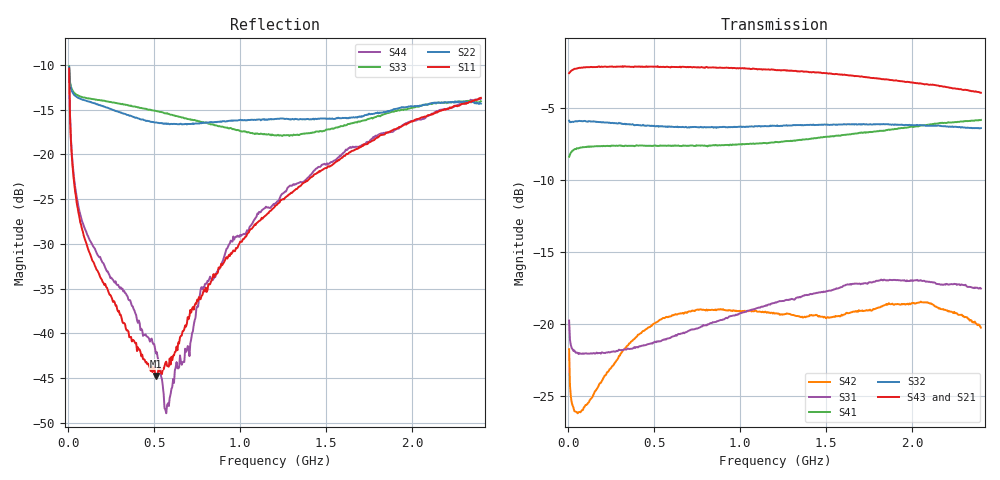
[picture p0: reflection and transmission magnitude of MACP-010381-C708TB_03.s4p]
!Agilent Technologies,E5071B,JP1KK00267,A.09.10
!Date: Mon Mar 23 11:06:01 2020
!Data & Calibration Information:
!DD.  Test Board PCB PT-0014848.  Pin Port mapping: Port1 – pin1, Port1 – pin2, Port3 – pin4, Port4 – pin5
!Freq	S11:SOLT4(ON)	S12:SOLT4(ON)	S13:SOLT4(ON)	S14:SOLT4(ON)
!	S21:SOLT4(ON)	S22:SOLT4(ON)	S23:SOLT4(ON)	S24:SOLT4(ON)
!	S31:SOLT4(ON)	S32:SOLT4(ON)	S33:SOLT4(ON)	S34:SOLT4(ON)
!	S41:SOLT4(ON)	S42:SOLT4(ON)	S43:SOLT4(ON)	S44:SOLT4(ON)
# Hz S MA R 75
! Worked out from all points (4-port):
!   480 points, 5 MHz to 2.4 GHz, reference 75 ohm
!   strongest paths, dB at 5 MHz, 605 MHz, 1.205 GHz, 1.805 GHz, 2.4 GHz:
!     S43: -2.5, -2.1, -2.3, -2.9, -3.9
!     S21: -2.6, -2.2, -2.4, -2.9, -3.8
!     S32: -5.9, -6.3, -6.2, -6.1, -6.4
!     S41: -8.4, -7.6, -7.3, -6.6, -5.8
!     S31: -19.7, -20.9, -18.5, -17.0, -17.5
!     S42: -21.7, -19.4, -19.2, -18.8, -20.2
!   lowest |S11| = -44.8 dB at 510 MHz (marker M1), VSWR 1.01, Z = 75.7 + j0.51 ohm
!   |S11| at or under -10 dB: start of sweep to end of sweep
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5000000  0.3027 111.4  0.7427 15.4  0.08397 154.5  0.3799 25.6
         0.7448 15.3  0.3089 143.8  0.5123 -172.0  0.09941 164.4
         0.1029 165.8  0.5099 -172.0  0.312 145.2  0.748 15.3
         0.3819 25.7  0.08191 153.2  0.7457 15.4  0.3033 113.3
1e8  0.03292 117.7  0.7791 -1.8  0.0514 167.4  0.4126 1.2
     0.7783 -2.0  0.2005 166.8  0.5098 173.0  0.07586 171.5
     0.07919 171.2  0.5084 172.8  0.2076 169.7  0.7833 -1.9
     0.413 1.1  0.05235 -176.3  0.7812 -1.8  0.03774 124.6
5.1e8  0.005769 35.7  0.7806 -16.5  0.06634 138.2  0.4181 -5.1
       0.78 -16.7  0.151 153.2  0.497 143.3  0.08616 144.6
       0.08654 144.7  0.487 142.5  0.1754 155.7  0.7909 -16.6
       0.4172 -4.9  0.1013 153.9  0.7854 -16.2  0.007706 82.3
5.75e8  0.006558 3.2  0.7812 -19.0  0.07058 133.1  0.4154 -5.7
        0.7771 -19.0  0.1481 153.2  0.4969 138.8  0.08878 140.2
        0.08917 140.1  0.4848 138.4  0.1702 153.5  0.7858 -18.9
        0.4175 -5.5  0.1059 145.5  0.7856 -18.6  0.003971 28.6
7.75e8  0.0162 -46.2  0.775 -26.0  0.08403 118.0  0.4155 -7.6
        0.7742 -25.7  0.1496 151.7  0.4936 125.3  0.09945 126.1
        0.09827 126.4  0.4837 125.3  0.1522 148.5  0.7829 -26.0
        0.4177 -7.5  0.1125 122.2  0.7832 -25.8  0.01809 -56.0
1.24e9  0.0556 -87.6  0.7542 -42.3  0.122 85.4  0.4313 -11.4
        0.7546 -42.4  0.1589 141.9  0.4902 94.5  0.1144 90.8
        0.1203 93.1  0.4893 94.6  0.1277 154.1  0.7653 -42.6
        0.4311 -11.4  0.1082 83.6  0.7632 -42.5  0.05961 -101.3
2.4e9  0.2075 -140.9  0.6442 -85.4  0.1404 13.0  0.5042 -29.7
       0.6489 -85.6  0.1928 118.9  0.479 15.7  0.09345 -6.3
       0.1331 10.5  0.4804 16.6  0.1987 146.6  0.6396 -87.3
       0.5128 -29.8  0.09727 -1.8  0.6375 -87.6  0.2051 -148.2
